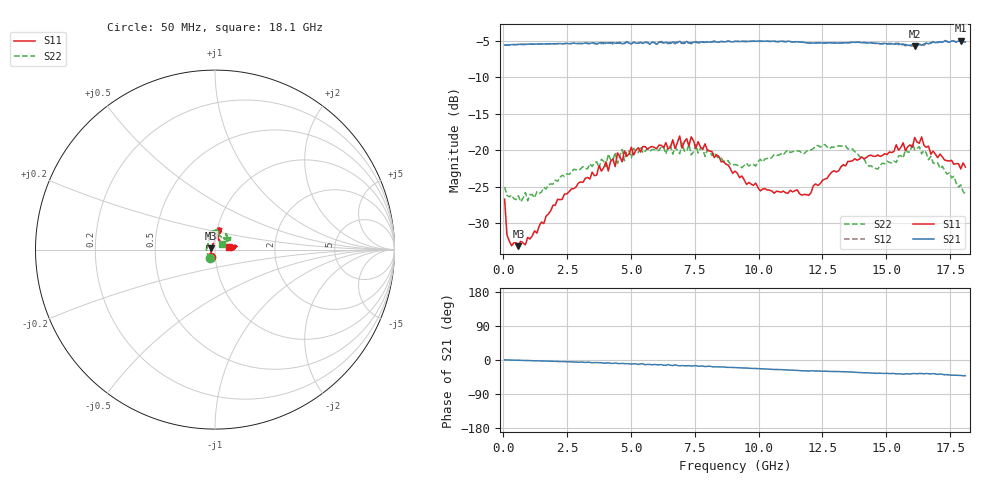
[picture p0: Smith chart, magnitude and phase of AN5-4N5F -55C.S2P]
! Network Analyzer HP8720D.06.14 Serial No. US36140669
! 28 Jun 2005  12:45:01
! Frequency  S11  S21  S12  S22
# HZ  S  DB R 50
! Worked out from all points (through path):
!   201 points, 50 MHz to 18.1 GHz, reference 50 ohm
!   highest |S21| = -5.01 dB at 17.92 GHz (marker M1); lowest = -5.7 dB at 16.11 GHz (marker M2)
!   group delay of S21, straight-line fit = 6.63 ps
!   lowest |S11| = -33.1 dB at 591.5 MHz (marker M3), VSWR 1.05, Z = 48 + j0.777 ohm
!   |S11| at or under -10 dB: start of sweep to end of sweep
!   |S22| runs from -27.1 to -19.0 dB; largest |S21 - S12| = 0.019
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5e7  -26.71 -116.0  -5.58 0.3  -5.60 0.2  -25.03 -120.9
1.4025e8  -31.55 -148.4  -5.61 0.2  -5.58 0.1  -26.15 -162.8
5.915e8  -33.13 158.5  -5.50 -0.5  -5.51 -0.6  -26.23 169.5
3.1185e9  -24.40 88.7  -5.38 -5.6  -5.41 -6.0  -22.24 119.1
4.021e9  -21.59 82.2  -5.31 -8.2  -5.39 -7.4  -22.23 109.5
4.382e9  -22.23 78.6  -5.35 -7.9  -5.31 -9.2  -20.29 108.8
4.47225e9  -20.36 74.4  -5.35 -9.1  -5.29 -8.2  -21.81 111.4
4.65275e9  -21.59 74.5  -5.42 -8.8  -5.25 -9.5  -19.90 109.9
4.743e9  -20.07 77.8  -5.38 -9.7  -5.37 -9.0  -21.43 105.5
6.09675e9  -19.30 75.9  -5.20 -12.7  -5.14 -12.7  -20.02 94.7
6.7285e9  -19.76 79.6  -5.23 -12.8  -5.41 -13.7  -19.54 87.5
6.909e9  -18.05 78.5  -5.07 -15.6  -5.19 -14.5  -20.47 85.0
6.99925e9  -19.71 77.6  -5.31 -14.5  -5.39 -15.9  -19.00 86.2
7.36025e9  -18.17 72.1  -5.41 -16.0  -5.24 -15.3  -20.64 89.3
7.54075e9  -19.73 71.7  -5.22 -14.9  -5.12 -16.7  -19.24 88.6
9.075e9  -22.84 77.6  -5.08 -20.0  -5.08 -20.1  -21.95 67.3
1.006775e10  -25.57 59.9  -5.04 -22.9  -5.10 -23.6  -21.23 50.9
1.21435e10  -24.84 27.8  -5.32 -28.5  -5.28 -28.8  -19.77 53.7
1.512175e10  -20.24 -1.2  -5.46 -35.9  -5.34 -36.0  -21.67 46.0
1.61145e10  -18.25 8.8  -5.71 -35.7  -5.46 -36.4  -19.95 39.7
1.79195e10  -22.56 10.8  -5.01 -40.8  -4.96 -40.9  -24.74 44.4
1.81e10  -22.30 10.6  -5.17 -41.5  -5.23 -42.0  -25.98 34.8
